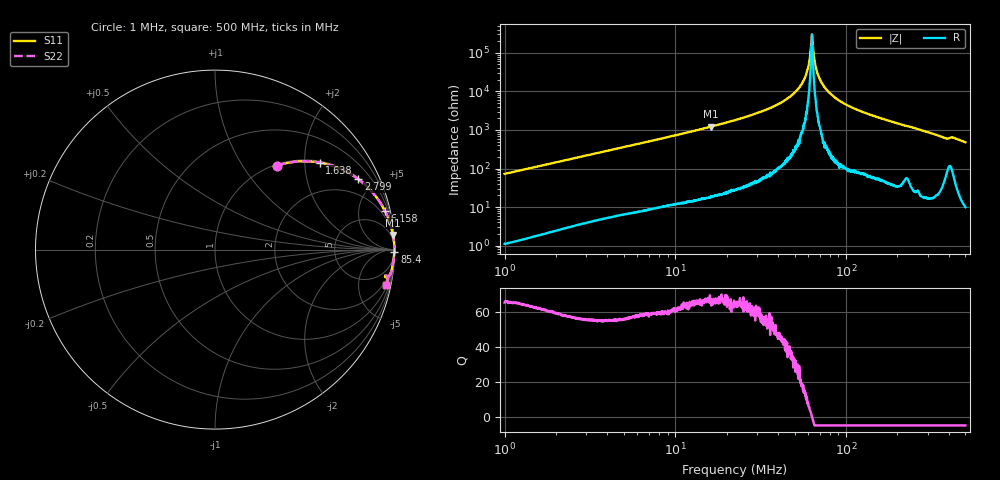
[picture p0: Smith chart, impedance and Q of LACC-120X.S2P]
!s-Parameter Generated by FASTRON Sdn. Bhd.
!FASTRON P/N : LACC-120X
!Keysight Technologies,E4991B,MY54100416,A.01.15
!Date: Wed Mar 18 09:28:24 2026
!Version  : Rev00 Wed Mar 18 09:28:24 2026
!Data & Calibration Information:
!PortZ  Port1:50+j0  Port2:50+j0
!When reading, reference impedance value at option line is always used.
!Remarks : This data is being provided solely for informational purposes.
!Freq	S11	S21	S12	S22
# Hz S dB R 50
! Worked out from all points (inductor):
!   1601 points, 1 MHz to 500 MHz, reference 50 ohm
!   read as one part in series: L = 11.5 uH near 1.032 MHz
!   highest Q = 67.3 at 16.14 MHz (marker M1), where L = 12 uH
!   self-resonance near 63.08 MHz
!   S11 on the Smith chart (normalised r, x): 1 MHz: 1.02, +1.45; 1.638 MHz: 1.04, +2.37; 2.799 MHz: 1.07, +4.03; 6.158 MHz: 1.15, +8.85; 85.4 MHz: open; 500 MHz: 1.20, -9.59
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1000000  -4.68 53.5  -1.90 -35.7  -1.90 -35.7  -4.68 53.5
1637686  -2.40 39.8  -3.88 -49.3  -3.88 -49.3  -2.40 39.8
2799090  -1.02 26.2  -7.11 -62.8  -7.11 -62.8  -1.02 26.2
2820919  -1.00 26.0  -7.16 -63.0  -7.16 -63.0  -1.00 26.0
6158128  -0.25 12.7  -13.16 -76.3  -13.16 -76.3  -0.25 12.7
7957584  -0.15 9.9  -15.33 -79.2  -15.33 -79.2  -0.15 9.9
1.613575e7  -0.04 4.7  -21.75 -84.5  -21.75 -84.5  -0.04 4.7
2.236068e7  -0.02 3.2  -25.11 -85.9  -25.11 -85.9  -0.02 3.2
3.676229e7  -0.01 1.5  -31.79 -87.4  -31.79 -87.4  -0.01 1.5
4.957817e7  -0.00 0.6  -39.06 -87.6  -39.06 -87.6  -0.00 0.6
5.746337e7  -0.00 0.2  -47.28 -85.9  -47.28 -85.9  -0.00 0.2
5.973923e7  -0.00 0.1  -51.86 -81.8  -51.86 -81.8  -0.00 0.1
6.186448e7  -0.00 0.1  -60.05 -71.2  -60.05 -71.2  -0.00 0.1
6.307767e7  -0.00 0.0  -69.54 -5.9  -69.54 -5.9  -0.00 0.0
6.431465e7  -0.00 -0.0  -61.65 68.8  -61.65 68.8  -0.00 -0.0
6.738328e7  -0.00 -0.2  -50.61 84.9  -50.61 84.9  -0.00 -0.2
7.032465e7  -0.00 -0.3  -46.14 86.4  -46.14 86.4  -0.00 -0.3
7.630124e7  -0.00 -0.5  -41.15 87.6  -41.15 87.6  -0.00 -0.5
8.539853e7  -0.00 -0.8  -37.01 88.0  -37.01 88.0  -0.00 -0.8
1.120806e8  -0.01 -1.6  -31.07 87.1  -31.07 87.1  -0.01 -1.6
1.77937e8  -0.03 -3.3  -24.82 85.4  -24.82 85.4  -0.03 -3.3
5e8  -0.22 -11.7  -13.84 77.1  -13.84 77.1  -0.22 -11.7
